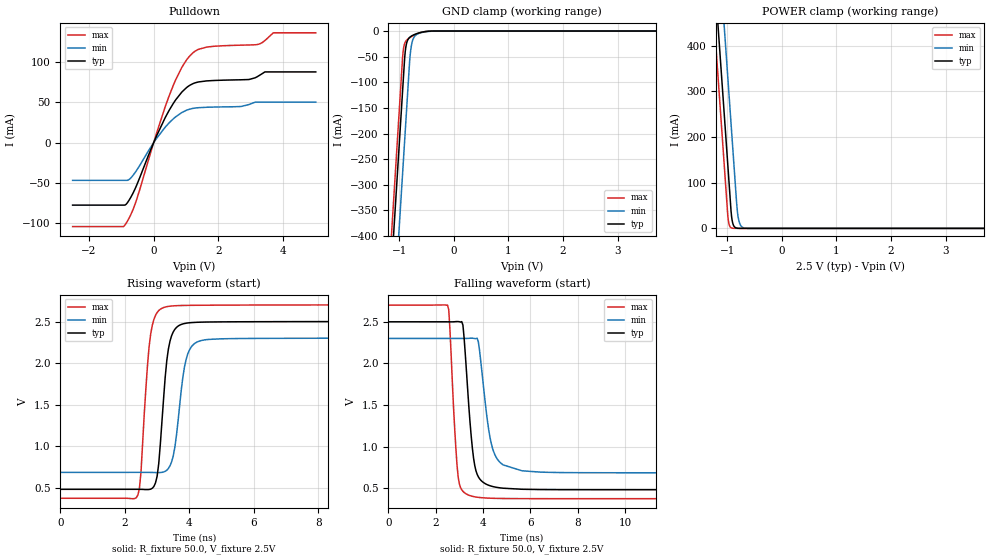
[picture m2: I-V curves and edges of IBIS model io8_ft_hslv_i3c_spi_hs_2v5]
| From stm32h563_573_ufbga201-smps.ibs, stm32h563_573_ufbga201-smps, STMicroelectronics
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[Model]   io8_ft_hslv_i3c_spi_hs_2v5
Model_type I/O_open_drain
Polarity   Non-Inverting
Enable   Active-Low
| CAP_THRESHOLD on pad IOFT is "UDTCAPC" :
| Rising=20.0% of vddiom   Falling=80.0% of vddiom
| C_comp min and max val. don't necessarily correlate with the min and max pvt
| but are the smallest and greatest pad capacitance found.
| var   typ   min   max
C_comp   3.87733pF  3.87281pF  3.96699pF
|C_comp_pulldown   3.87733pF  3.87281pF  3.96699pF
Vinl = 1.15V
Vinh = 1.35V
Vmeas = 1.25V   | Reference voltage for timing measurements
Cref  = 50.0pF   | Timing specification test load capacitance value
Rref  = 1.0MOhm   | Timing specification test load resistance value
Vref  = 1.375V   | Timing specification test load voltage
[Model Spec]
| TIME_THRESHOLD on pin ZII2CV11 is "CMOS" :
| Rising=40.0% of vdd   Falling=60.0% of vdd
Vinl 989.80000mV 917.80000mV 1.06580V
Vinh 1.40320V 1.29620V 1.49120V
| variable   typ   min   max
[Temperature Range] 25.0 125.0 -40.0
| variable   typ   min   max
[Voltage Range] 2.5V 2.3V 2.7V
| variable   typ   min   max
[POWER Clamp Reference] 2.5V 2.3V 2.7V
| variable   typ   min   max
[GND Clamp Reference] 0V 0V 0V
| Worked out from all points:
|   slope of the pulldown table from 0 to 0.375 V, typ, clamps not added: 11.5 ohm
|   GND clamp passes 1 mA (typ) near -0.52 V on its own axis
|   POWER clamp passes 1 mA (typ) near -0.84 V on its own axis
|   rising waveform, R_fixture 50.0, V_fixture 2.5V: 20-80 % time 254ps typ, 305ps min, 242ps max; typ from 0.481 V to 2.5 V
|   falling waveform, R_fixture 50.0, V_fixture 2.5V: 20-80 % time 336ps typ, 452ps min, 255ps max; typ from 2.5 V to 0.481 V
[POWER Clamp]
-2.5V     2.708A     2.899A     2.597A
-1.23V    548.8mA    740.2mA    437.5mA
-1.16V    429.8mA    621.2mA    318.5mA
-1.12V    361.8mA    553.2mA    250.5mA
-1.03V    208.8mA    400.2mA    97.53mA
-980mV    123.8mA    315.2mA    17.95mA
-920mV    26.3mA     213.2mA    906uA
-880mV    5.543mA    145.2mA    123.7uA
-810mV    363.5uA    33.6mA     3.797uA
-770mV    76.62uA    10.47mA    518.8nA
-700mV    5.026uA    1.361mA    16.11nA
5V        0A         0A         0A
[GND Clamp]
-2.5V     -2.77A     -2.931A    -2.704A
-1.21V    -576.8mA   -738.1mA   -511.3mA
-950mV    -134.8mA   -296.1mA   -69.34mA
-920mV    -83.82mA   -245.1mA   -32.48mA
-900mV    -50.56mA   -211.1mA   -24.02mA
-880mV    -31.31mA   -177.1mA   -19.85mA
-850mV    -18.7mA    -126.1mA   -16.34mA
-800mV    -11.46mA   -46.18mA   -12.45mA
-750mV    -8.203mA   -16.63mA   -9.325mA
-650mV    -4.063mA   -4.987mA   -4.427mA
-360mV    -35.05uA   -165.1uA   -9.564uA
5V        7.96nA     1.281uA    294pA
| variable   typ   min   max
[Pullup Reference] 2.5V 2.3V 2.7V
| variable   typ   min   max
[Pulldown Reference] 0V 0V 0V
[Pulldown]
-2.5V     -77.63mA   -46.85mA   -104.3mA
-870mV    -77.24mA   -46.85mA   -101.4mA
-550mV    -55.3mA    -35.88mA   -73.72mA
90mV      8.401mA    5.299mA    11.79mA
610mV     49.03mA    29.76mA    71.69mA
870mV     62.92mA    37.48mA    93.62mA
1.23V     73.63mA    42.72mA    112.2mA
1.64V     76.78mA    44.01mA    118.8mA
2.7V      78.15mA    44.99mA    121.2mA
3.22V     82.58mA    50.35mA    122.2mA
3.69V     87.93mA    50.35mA    136.5mA
5V        87.93mA    50.35mA    136.5mA
[Ramp]
dV/dt_r 1.21161V/249.77465ps 969.20766mV/302.74296ps 1.39625V/238.72272ps
dV/dt_f 1.21165V/334.8567ps 969.26185mV/450.62736ps 1.39628V/253.2706ps
R_load = 50.0
| Removed startup time: 0s 0s 0s  .
| Removed end time: 24.4ns.
[Rising Waveform]
R_fixture   = 50.0
V_fixture   = 2.5V
V_fixture_min = 2.3V
V_fixture_max = 2.7V
0s        480.6mV    684.6mV    372.9mV
2.4ns     480.5mV    684.8mV    408.9mV
2.5ns     480.2mV    684.8mV    692mV
2.8ns     482.7mV    684mV      2.35V
3ns       638mV      681.9mV    2.609V
3.25ns    1.828V     697.1mV    2.674V
3.5ns     2.375V     882.2mV    2.689V
3.9ns     2.48V      2.044V     2.694V
4.4ns     2.493V     2.274V     2.696V
24.4ns    2.5V       2.3V       2.7V
| Removed startup time: 0s 0s 0s  .
| Removed end time: 39.4ns.
[Falling Waveform]
R_fixture   = 50.0
V_fixture   = 2.5V
V_fixture_min = 2.3V
V_fixture_max = 2.7V
0s        2.5V       2.3V       2.7V
2.5ns     2.5V       2.3V       2.701V
2.55ns    2.5V       2.3V       2.646V
2.95ns    2.503V     2.3V       632.2mV
3.15ns    2.461V     2.3V       461.6mV
3.6ns     859.6mV    2.301V     398.4mV
3.8ns     636.6mV    2.262V     389mV
4.45ns    516.5mV    936.6mV    377.5mV
5.65ns    486.3mV    708.2mV    373.6mV
39.4ns    480.6mV    684.6mV    372.9mV
